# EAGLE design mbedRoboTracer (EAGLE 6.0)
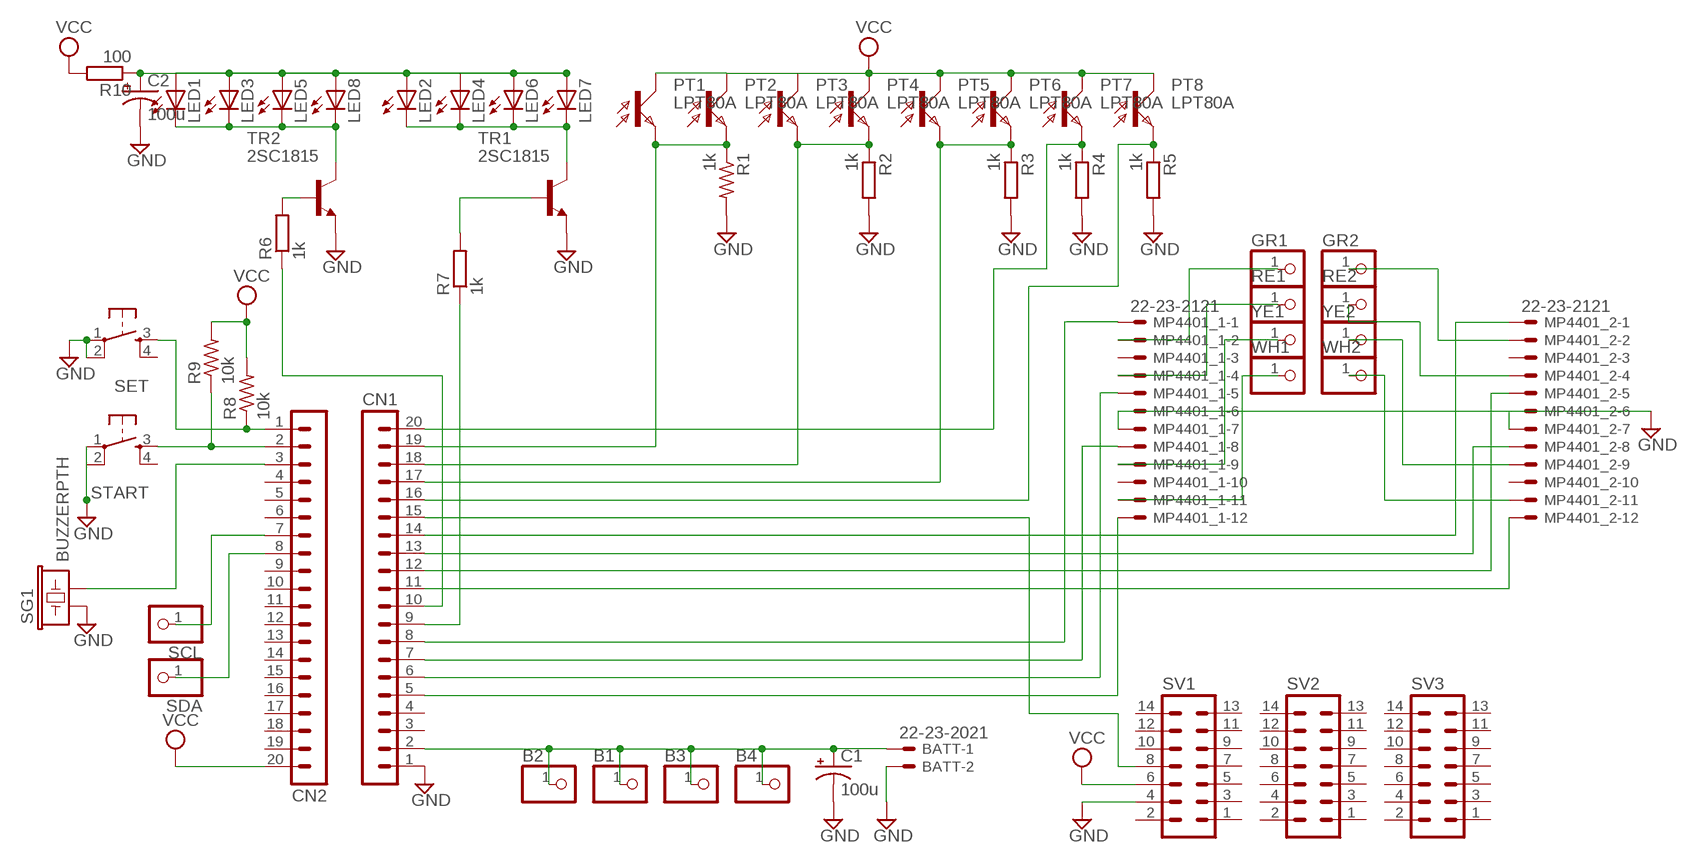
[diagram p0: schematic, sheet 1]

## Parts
B1  PINHD-1X1  [1X01]
B2  PINHD-1X1  [1X01]
B3  PINHD-1X1  [1X01]
B4  PINHD-1X1  [1X01]
BATT  22-23-2021  [22-23-2021]
C1  100u  CPOL-USTT2D5  [TT2D5]
C2  100u  CPOL-USTT2D5  [TT2D5]
CN1  MA20-1  [MA20-1]
CN2  MA20-1  [MA20-1]
GR1  PINHD-1X1  [1X01]
GR2  PINHD-1X1  [1X01]
LED1  LED3MM  [LED3MM]
LED2  LED3MM  [LED3MM]
LED3  LED3MM  [LED3MM]
LED4  LED3MM  [LED3MM]
LED5  LED3MM  [LED3MM]
LED6  LED3MM  [LED3MM]
LED7  LED3MM  [LED3MM]
LED8  LED3MM  [LED3MM]
MP4401_1  22-23-2121  [22-23-2121]
MP4401_2  22-23-2121  [22-23-2121]
PT1  LPT80A  [LPT80A]
PT2  LPT80A  [LPT80A]
PT3  LPT80A  [LPT80A]
PT4  LPT80A  [LPT80A]
PT5  LPT80A  [LPT80A]
PT6  LPT80A  [LPT80A]
PT7  LPT80A  [LPT80A]
PT8  LPT80A  [LPT80A]
R1  1k  R-US_0204/2V  [0204V]
R2  1k  R-EU_0204/2V  [0204V]
R3  1k  R-EU_0204/2V  [0204V]
R4  1k  R-EU_0204/2V  [0204V]
R5  1k  R-EU_0204/2V  [0204V]
R6  1k  R-EU_0204/2V  [0204V]
R7  1k  R-EU_0204/2V  [0204V]
R8  10k  R-US_0204/2V  [0204V]
R9  10k  R-US_0204/2V  [0204V]
R10  100  R-EU_0204/2V  [0204V]
RE1  PINHD-1X1  [1X01]
RE2  PINHD-1X1  [1X01]
SCL  PINHD-1X1  [1X01]
SDA  PINHD-1X1  [1X01]
SET  T-SWITCH-10  [B3F-10XX]
SG1  BUZZERPTH  [BUZZER-12MM]
START  T-SWITCH-10  [B3F-10XX]
SV1  MA07-2  [MA07-2]
SV2  MA07-2  [MA07-2]
SV3  MA07-2  [MA07-2]
TR1  2SC1815  [TO92-ECB]
TR2  2SC1815  [TO92-ECB]
WH1  PINHD-1X1  [1X01]
WH2  PINHD-1X1  [1X01]
YE1  PINHD-1X1  [1X01]
YE2  PINHD-1X1  [1X01]

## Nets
GND: BATT.2 C1.- C2.- CN1.1 MP4401_1.6 MP4401_1.7 MP4401_2.6 MP4401_2.7 R1.2 R2.2 R3.2 R4.2 R5.2 SET.1(P) SET.2(P1) SG1.+ START.1(P) START.2(P1) SV1.4 TR1.E TR2.E
N$1: CN1.17 PT5.E PT6.E R3.1
N$2: R7.2 TR1.B
N$3: CN1.8 MP4401_1.1
N$4: CN2.2 R9.1 START.3(S)
N$5: CN2.1 R8.1 SET.3(S)
N$6: CN1.15 SV1.8
N$7: LED1.K(C) LED3.K(C) LED5.K(C) LED8.K(C) TR2.C
N$8: CN1.18 PT3.E PT4.E R2.1
N$9: CN2.7 SCL.1
N$10: CN2.8 SDA.1
N$11: C2.+ LED1.A LED2.A LED3.A LED4.A LED5.A LED6.A LED7.A LED8.A R10.1
N$16: CN1.11 MP4401_2.12
N$17: CN1.6 MP4401_1.5
N$18: LED2.K(C) LED4.K(C) LED6.K(C) LED7.K(C) TR1.C
N$19: R6.2 TR2.B
N$20: CN2.3 SG1.-
N$21: CN1.20 PT7.E R4.1
N$22: CN1.9 R7.1
N$24: CN1.19 PT1.E PT2.E R1.1
N$25: B1.1 B2.1 B3.1 B4.1 BATT.1 C1.+ CN1.2
N$26: CN1.16 PT8.E R5.1
N$28: CN1.14 MP4401_2.1
N$29: CN1.10 R6.1
N$39: CN1.7 MP4401_1.8
N$41: CN1.12 MP4401_2.5
N$44: GR1.1 MP4401_1.2
N$45: MP4401_1.4 RE1.1
N$46: MP4401_1.11 WH1.1
N$47: CN1.5 MP4401_1.12
N$48: GR2.1 MP4401_2.2
N$49: MP4401_2.4 RE2.1
N$50: MP4401_2.9 YE2.1
N$51: MP4401_2.11 WH2.1
N$52: MP4401_1.9 YE1.1
N$61: CN1.13 MP4401_2.8
VCC: CN2.20 PT1.C PT2.C PT3.C PT4.C PT5.C PT6.C PT7.C PT8.C R8.2 R9.2 R10.2 SV1.6
Unconnected: CN1.3 CN1.4 CN2.4 CN2.5 CN2.6 CN2.9 CN2.10 CN2.11 CN2.12 CN2.13 CN2.14 CN2.15 CN2.16 CN2.17 CN2.18 CN2.19 MP4401_1.3 MP4401_1.10 MP4401_2.3 MP4401_2.10 SET.4(S1) START.4(S1) SV1.1 SV1.2 SV1.3 SV1.5 SV1.7 SV1.9 SV1.10 SV1.11 SV1.12 SV1.13 SV1.14 SV2.1 SV2.2 SV2.3 SV2.4 SV2.5 SV2.6 SV2.7 SV2.8 SV2.9 SV2.10 SV2.11 SV2.12 SV2.13 SV2.14 SV3.1 SV3.2 SV3.3 SV3.4 SV3.5 SV3.6 SV3.7 SV3.8 SV3.9 SV3.10 SV3.11 SV3.12 SV3.13 SV3.14

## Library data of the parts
B1-B4 GR1 GR2 RE1 RE2 SCL SDA WH1 WH2 YE1 YE2 = pinhead:PINHD-1X1: PIN HEADER
BATT = con-molex:22-23-2021: .100" (2.54mm) Center Header - 2 Pin
C1 C2 = resistor:CPOL-US: POLARIZED CAPACITOR, American symbol
CN1 CN2 = con-lstb:MA20-1: PIN HEADER; OC_FARNELL: unknown; OC_NEWARK: unknown
LED1-LED8 = led:LED: LED
MP4401_1 MP4401_2 = con-molex:22-23-2121: .100" (2.54mm) Center Header - 12 Pin
PT1-PT8 = opto-trans-siemens:LPT80A: PHOTO TRANSISTOR
R1 R8 R9 = resistor:R-US_: RESISTOR, American symbol
R2-R7 = rcl:R-EU_: RESISTOR, European symbol
R10 = resistor:R-EU_: RESISTOR, European symbol
SET START = 1-sw:T-SWITCH: TACTILE SWITCH
SG1 = SparkFun:BUZZER: Buzzer 12mm
SV1-SV3 = con-lstb:MA07-2: PIN HEADER; OC_FARNELL: unknown; OC_NEWARK: unknown
TR1 TR2 = transistor:2SC1815: NPN EPITAXIAL TRANSISTOR Source: TOSHIBA .. 2SC1815 1.pdf

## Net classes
1 +5V: width 0.61 mm, drill 0.406 mm
2 GND: width 0.914 mm, drill 0.406 mm

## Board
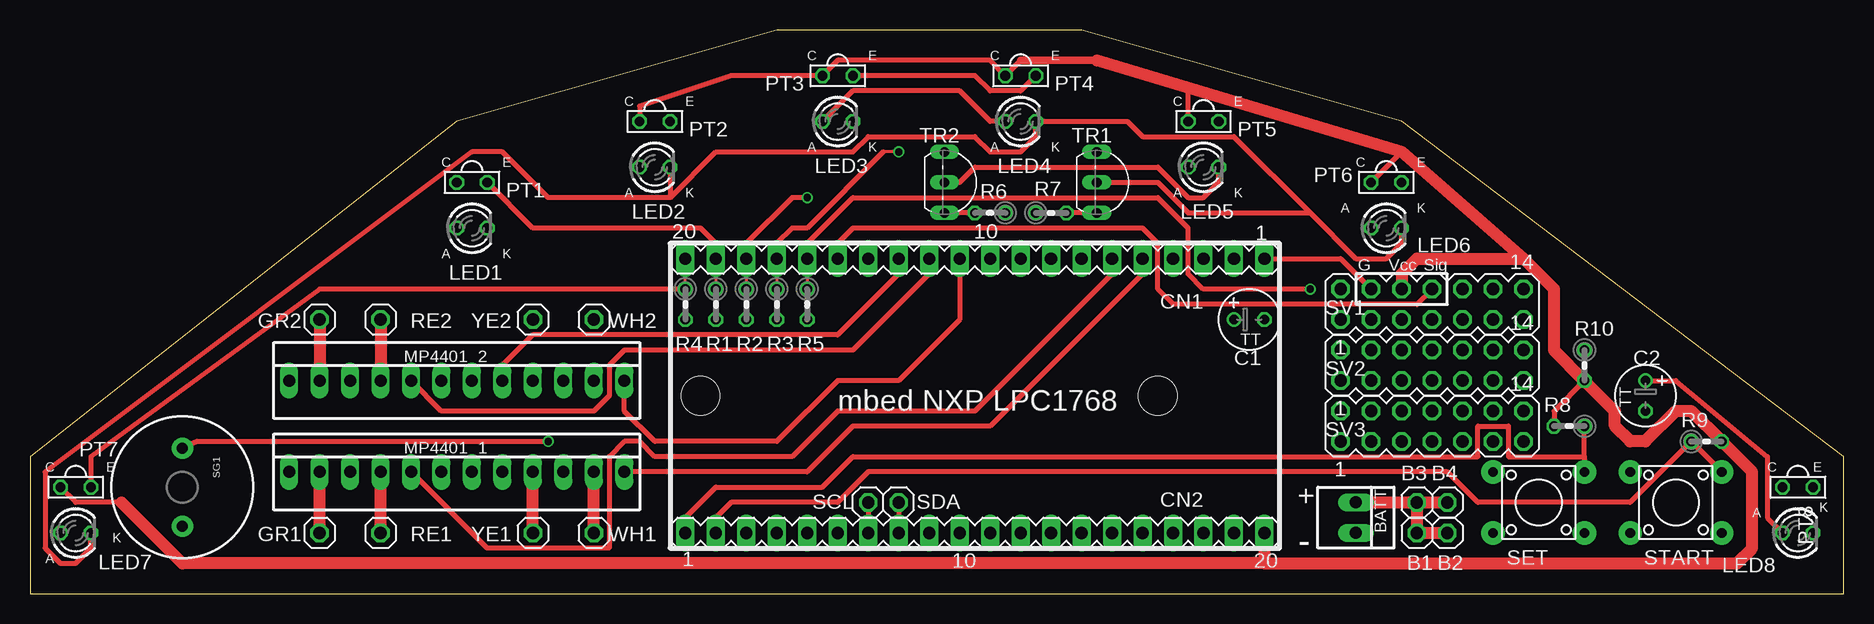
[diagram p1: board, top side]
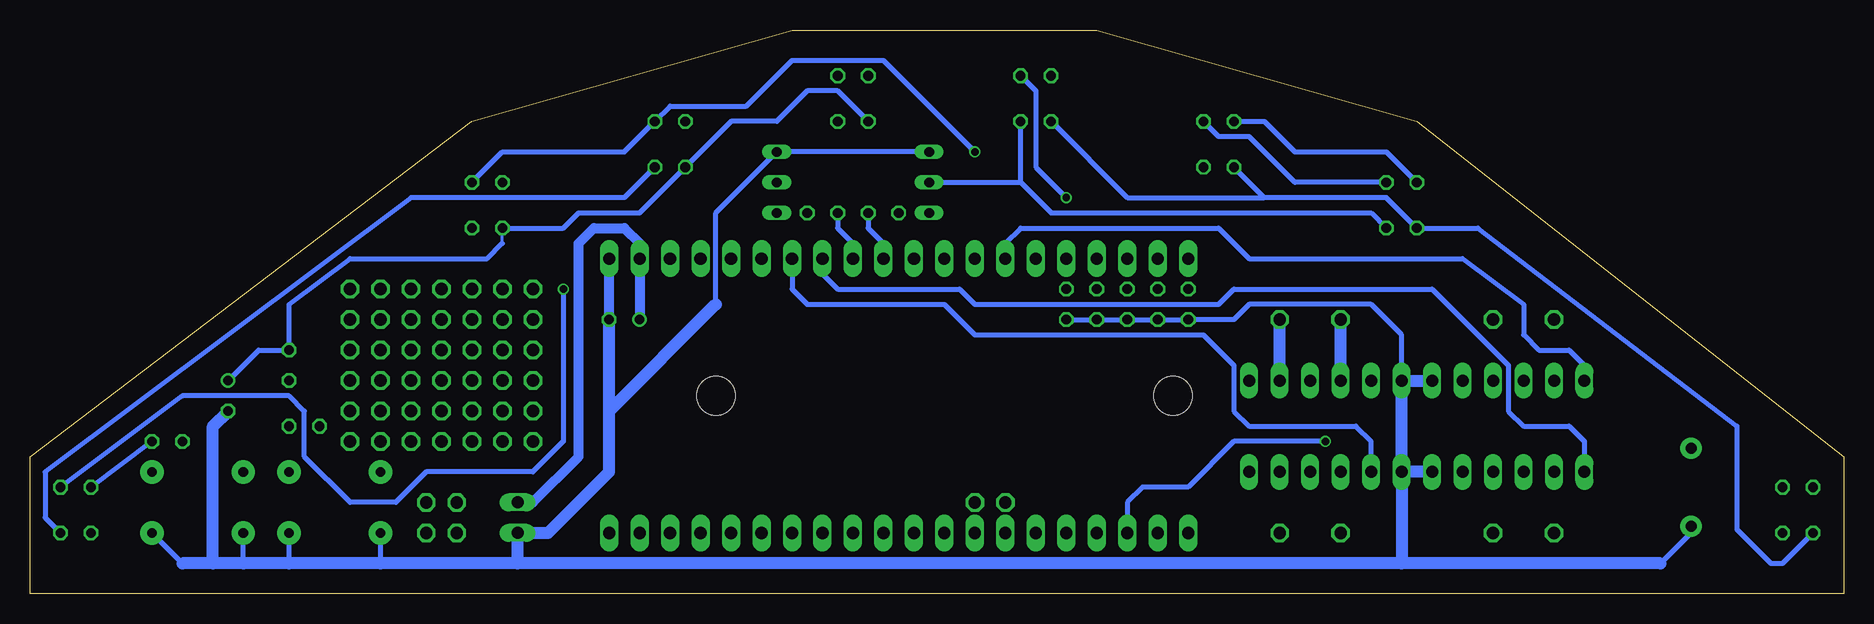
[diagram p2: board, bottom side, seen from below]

Size 151.13 x 46.99 mm. Coordinates in mm from the lower left corner, seen from the top.
Outline: 0,0 151.13,0 151.13,11.43 114.3,39.37 87.63,46.99 62.23,46.99 35.56,39.37 0,11.43 0,0
Copper layers (1*16): Top 0.035mm / dielectric 1.53mm / Bottom 0.035mm
Design rules: minimum track width 5mil, minimum drill 0.3mm, track to track 5mil, track to pad 0.229mm, pad to pad 5mil, via to via 5mil, smd to smd 5mil, copper to edge 0.5mm, drill to drill 0.5mm, minimum pad ring 0.15mm, minimum via ring 0.15mm, stop-mask expansion 4mil, vias tented up to drill 0.35mm, thermal gap 10mil
Holes 3.2 mm at 55.88,16.51 93.98,16.51

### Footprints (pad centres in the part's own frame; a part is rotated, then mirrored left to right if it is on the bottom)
1X01 = drill 1.016 octagon: 1 0,0
22-23-2021 = drill 1 long: 1 -1.27,0; 2 1.27,0
TT2D5 = drill 0.813: + -1.27,0 | drill 0.813 octagon: - 1.27,0
MA20-1 = drill 1.016 long: 1 -24.13,0; 2 -21.59,0; 3 -19.05,0; 4 -16.51,0; 5 -13.97,0; 6 -11.43,0; 7 -8.89,0; 8 -6.35,0; 9 -3.81,0; 10 -1.27,0; 11 1.27,0; 12 3.81,0; 13 6.35,0; 14 8.89,0; 15 11.43,0; 16 13.97,0; 17 16.51,0; 18 19.05,0; 19 21.59,0; 20 24.13,0
LED3MM = drill 0.813 octagon: A -1.27,0; K 1.27,0
22-23-2121 = drill 1 long: 1 -13.97,0; 2 -11.43,0; 3 -8.89,0; 4 -6.35,0; 5 -3.81,0; 6 -1.27,0; 7 1.27,0; 8 3.81,0; 9 6.35,0; 10 8.89,0; 11 11.43,0; 12 13.97,0
LPT80A = drill 0.813 octagon: C 0,-1.27; E 0,1.27
0204V = drill 0.813 octagon: 1 -1.27,0; 2 1.27,0
B3F-10XX = drill 0.813 pad 1.93: 1 -3.81,2.54; 2 3.81,2.54; 3 -3.81,-2.54; 4 3.81,-2.54
BUZZER-12MM = drill 0.9 pad 1.778: + 3.25,0; - -3.25,0
MA07-2 = drill 1.016 octagon: 1 -7.62,-1.27; 2 -7.62,1.27; 3 -5.08,-1.27; 4 -5.08,1.27; 5 -2.54,-1.27; 6 -2.54,1.27; 7 0,-1.27; 8 0,1.27; 9 2.54,-1.27; 10 2.54,1.27; 11 5.08,-1.27; 12 5.08,1.27; 13 7.62,-1.27; 14 7.62,1.27
TO92-ECB = drill 0.813 long: B 2.54,0; C 0,0; E -2.54,0

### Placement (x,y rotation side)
B1  115.57,5.08 0 top
B2  115.57,7.62 0 top
B3  118.11,7.62 0 top
B4  118.11,5.08 0 top
BATT  110.49,6.35 270 top
C1  101.6,22.86 0 top
C2  134.62,16.51 270 top
CN1  78.74,27.94 180 top
CN2  78.74,5.08 0 top
GR1  24.13,5.08 0 top
GR2  24.13,22.86 0 top
LED1  36.83,30.48 0 top
LED2  52.07,35.56 0 top
LED3  67.31,39.37 0 top
LED4  82.55,39.37 0 top
LED5  97.79,35.56 0 top
LED6  113.03,30.48 0 top
LED7  3.81,5.08 0 top
LED8  147.32,5.08 0 top
MP4401_1  35.56,10.16 0 top
MP4401_2  35.56,17.78 0 top
PT1  36.83,34.29 270 top
PT2  52.07,39.37 270 top
PT3  67.31,43.18 270 top
PT4  82.55,43.18 270 top
PT5  97.79,39.37 270 top
PT6  113.03,34.29 270 top
PT7  3.81,8.89 270 top
PT8  147.32,8.89 270 top
R1  57.15,24.13 270 top
R2  59.69,24.13 270 top
R3  62.23,24.13 270 top
R4  54.61,24.13 270 top
R5  64.77,24.13 270 top
R6  80.01,31.75 180 top
R7  85.09,31.75 0 top
R8  128.27,13.97 180 top
R9  139.7,12.7 0 top
R10  129.54,19.05 270 top
RE1  29.21,5.08 0 top
RE2  29.21,22.86 0 top
SCL  69.85,7.62 180 top
SDA  72.39,7.62 180 top
SET  125.73,7.62 180 top
SG1  12.7,8.89 270 top
START  137.16,7.62 180 top
SV1  116.84,24.13 0 top
SV2  116.84,19.05 0 top
SV3  116.84,13.97 0 top
TR1  88.9,34.29 270 top
TR2  76.2,34.29 270 top
WH1  46.99,5.08 0 top
WH2  46.99,22.86 0 top
YE1  41.91,5.08 0 top
YE2  41.91,22.86 0 top

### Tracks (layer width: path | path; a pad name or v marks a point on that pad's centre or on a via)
GND
  Top 0.406: CN1.1 109.22,27.94 SV1.4
  Bottom 0.406: SG1.+ 12.7,5.08 15.24,2.54 | 138.43,2.54 START.1 | 121.92,2.54 SET.2 | 129.54,2.54 SET.1 | 133.35,2.54 START.2 | MP4401_2.7 36.83,21.59 39.37,24.13 49.53,24.13 50.8,22.86 R4.2 R1.2 R2.2 R3.2 R5.2 | 93.98,24.13 93.98,31.75 TR1.E TR2.E
  Bottom 0.813: C1.- CN1.1
  Bottom 1.016: 102.87,15.24 102.87,10.16 107.95,5.08 BATT.2 110.49,2.54 | 102.87,15.24 C1.- | 15.24,2.54 36.83,2.54 | 36.83,2.54 110.49,2.54 | 110.49,2.54 121.92,2.54 129.54,2.54 133.35,2.54 135.89,2.54 | 135.89,2.54 138.43,2.54 | MP4401_1.7 36.83,2.54 | 102.87,15.24 93.98,24.13 | 135.89,2.54 135.89,13.97 C2.- | MP4401_2.6 MP4401_2.7 MP4401_1.7 | MP4401_1.6 MP4401_1.7
N$1  (via drill 0.61)
  Top 0.254: CN1.17 R3.1 | v72.39,36.83 71.12,36.83
  Top 0.406: 71.12,36.83 64.77,30.48 63.5,30.48 62.23,29.21 CN1.17
  Bottom 0.406: PT6.E 111.76,36.83 101.6,36.83 PT5.E 97.79,40.64 91.44,40.64 87.63,44.45 80.01,44.45 v72.39,36.83
N$2
  Top 0.406: TR1.B R7.2
N$3
  Bottom 0.254: CN1.8 85.09,26.67
  Bottom 0.406: MP4401_1.1 21.59,12.7 22.86,13.97 26.67,13.97 27.94,15.24 27.94,19.05 34.29,25.4 50.8,25.4 52.07,24.13 72.39,24.13 73.66,25.4 83.82,25.4 85.09,26.67
N$4
  Top 0.254: 57.15,6.35 CN2.2
  Top 0.406: START.3 R9.1 133.35,7.62 120.65,7.62 118.11,10.16 69.85,10.16 67.31,7.62 58.42,7.62 57.15,6.35
N$5
  Top 0.254: 54.61,6.35 CN2.1
  Top 0.406: 54.61,6.35 57.15,8.89 66.04,8.89 68.58,11.43 120.65,11.43 120.65,13.97 123.19,13.97 123.19,11.43 129.54,11.43 | 129.54,11.43 R8.1 | 129.54,11.43 SET.3
N$6
  Top 0.406: CN1.15 67.31,29.21 68.58,30.48 92.71,30.48 93.98,29.21 93.98,25.4 95.25,24.13 115.57,24.13 SV1.8
N$7
  Top 0.406: TR2.C 77.47,34.29 78.74,35.56 93.98,35.56 96.52,33.02 97.79,33.02 99.06,34.29 LED5.K
  Bottom 0.406: LED1.K 39.37,31.75 66.04,31.75 68.58,34.29 | TR2.C 68.58,34.29 | 68.58,34.29 LED3.K | LED5.K 101.6,33.02 119.38,33.02 149.86,10.16 149.86,6.35 LED8.K
N$8  (via drill 0.61)
  Top 0.254: CN1.18 R2.1
  Top 0.406: PT3.E 78.74,43.18 80.01,41.91 82.55,41.91 PT4.E | v64.77,33.02 63.5,33.02 59.69,29.21 CN1.18
  Bottom 0.406: v64.77,33.02 67.31,35.56 67.31,41.91 PT3.E
N$9
  Top 0.406: SCL.1 CN2.7
N$10
  Top 0.406: SDA.1 CN2.8
N$11
  Top 0.406: LED8.A 144.78,6.35 144.78,11.43 137.16,17.78 C2.+ | LED3.A 68.58,41.91 77.47,41.91 80.01,39.37 LED4.A
  Bottom 0.254: 111.76,29.21 LED6.A
  Bottom 0.406: 48.26,33.02 59.69,33.02 LED3.A | LED7.A 5.08,2.54 6.05,2.54 8.89,5.38 8.89,13.97 30.48,30.48 LED1.A 38.1,33.02 48.26,33.02 | 48.26,33.02 LED2.A | 111.76,29.21 113.03,27.94 124.46,27.94 129.54,24.13 R10.1 132.08,20.32 C2.+ | LED6.A 106.68,30.48 105.41,31.75 100.33,31.75 LED5.A 92.71,39.37 88.9,39.37 86.36,41.91 83.82,41.91 LED4.A
N$16
  Top 0.406: CN1.11 77.47,22.86 72.39,17.78 67.31,17.78 62.23,12.7 52.07,12.7 49.53,15.24 MP4401_2.12
N$17
  Top 0.406: MP4401_1.5 38.1,3.81 48.26,3.81 48.26,11.43 49.53,12.7 50.8,12.7 52.07,11.43 63.5,11.43 67.31,15.24 78.74,15.24 90.17,26.67 CN1.6
N$18
  Top 0.406: LED2.K 53.34,33.02 | 53.34,33.02 43.18,33.02 39.37,36.83 36.83,36.83 1.27,10.16 1.27,3.81 2.54,2.54 3.81,2.54 5.08,3.81 LED7.K | 53.34,33.02 57.15,36.83 68.58,36.83 69.85,38.1 78.74,38.1 80.01,36.83 82.55,36.83 83.82,38.1 LED4.K 91.44,39.37 92.71,38.1 100.33,38.1 106.68,31.75 | LED6.K 114.3,29.21 113.03,27.94 110.49,27.94 106.68,31.75 | TR1.C 93.98,34.29 96.52,31.75 106.68,31.75
N$19
  Top 0.406: R6.2 TR2.B
N$20  (via drill 0.61)
  Top 0.406: v43.18,12.7 13.97,12.7 SG1.-
  Bottom 0.406: v43.18,12.7 50.8,12.7 54.61,8.89 58.42,8.89 59.69,7.62 CN2.3
N$21
  Top 0.254: R4.1 CN1.20
  Top 0.406: PT7.E 5.08,11.43 24.13,25.4 R4.1
N$22
  Bottom 0.406: R7.1 83.82,30.48 82.55,29.21 CN1.9
N$24
  Top 0.254: CN1.19 R1.1
  Top 0.406: PT1.E 41.91,30.48 55.88,30.48 57.15,29.21 CN1.19
  Bottom 0.406: PT2.E 52.07,38.1 49.53,38.1 45.72,34.29 PT1.E
N$25
  Top 1.016: B2.1 B1.1 B4.1 | B2.1 B3.1 | BATT.1 B2.1
  Bottom 0.406: BATT.1 109.22,7.62
  Bottom 0.813: 109.22,7.62 105.41,11.43 105.41,29.21 104.14,30.48 101.6,30.48 100.33,29.21 CN1.2 C1.+
N$26  (via drill 0.61)
  Top 0.254: R5.1 CN1.16 64.77,29.21
  Top 0.406: v106.68,25.4 97.79,25.4 96.52,26.67 96.52,30.48 93.98,33.02 68.58,33.02 64.77,29.21
  Bottom 0.406: PT8.E 138.43,16.51 129.54,16.51 128.27,15.24 128.27,11.43 124.46,7.62 120.65,7.62 118.11,10.16 109.22,10.16 106.68,12.7 v106.68,25.4
N$28
  Bottom 0.254: CN1.14 69.85,29.21
  Bottom 0.406: MP4401_2.1 21.59,19.05 22.86,20.32 25.4,20.32 26.67,21.59 26.67,24.13 31.75,27.94 49.53,27.94 52.07,30.48 68.58,30.48 69.85,29.21
N$29
  Bottom 0.406: R6.1 81.28,30.48 80.01,29.21 CN1.10
N$39
  Bottom 0.406: CN1.7 87.63,25.4 86.36,24.13 74.93,24.13 72.39,21.59 53.34,21.59 50.8,19.05 50.8,15.24 49.53,13.97 40.64,13.97 39.37,12.7 MP4401_1.8
N$41
  Top 0.254: CN1.12 74.93,26.67
  Top 0.406: MP4401_2.5 34.29,15.24 46.99,15.24 48.26,16.51 48.26,19.05 49.53,20.32 68.58,20.32 74.93,26.67
N$44
  Top 1.016: GR1.1 MP4401_1.2
N$45
  Top 1.016: RE1.1 MP4401_1.4
N$46
  Top 1.016: WH1.1 MP4401_1.11
N$47
  Top 0.406: MP4401_1.12 64.77,10.16 68.58,13.97 80.01,13.97 92.71,26.67 CN1.5
N$48
  Top 1.016: GR2.1 MP4401_2.2
N$49
  Top 1.016: RE2.1 MP4401_2.4
N$50
  Bottom 1.016: MP4401_2.9 YE2.1
N$51
  Bottom 1.016: MP4401_2.11 WH2.1
N$52
  Top 1.016: YE1.1 MP4401_1.9
N$61
  Top 0.254: CN1.13 72.39,26.67
  Top 0.406: MP4401_2.8 39.37,19.05 41.91,21.59 67.31,21.59 72.39,26.67
VCC
  Top 0.406: 88.9,44.45 96.52,41.91 PT5.C | PT2.C 50.8,40.64 58.42,43.18 PT3.C 67.31,44.45 80.01,44.45 PT4.C 82.55,44.45 | PT7.C 3.81,7.62 7.62,7.62 | R10.2 127,15.24 R8.2 | 114.3,36.83 PT6.C
  Top 0.61: 82.55,44.45 88.9,44.45
  Top 1.016: CN2.20 102.87,2.54 | 7.62,7.62 12.7,2.54 102.87,2.54 | 102.87,2.54 142.24,2.54 143.51,3.81 143.51,10.16 R9.2 138.43,15.24 137.16,15.24 134.62,12.7 133.35,12.7 132.08,13.97 132.08,15.24 R10.2 127,20.32 127,25.4 124.46,27.94 | 88.9,44.45 114.3,36.83 124.46,27.94 | 124.46,27.94 115.57,27.94 114.3,26.67 SV1.6
  Bottom 0.406: PT1.C 38.1,36.83 45.72,36.83 48.26,39.37 PT2.C | PT8.C R9.2

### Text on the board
tPlace: C | E | C | E | C | E | C | E | A | K | A | K | C | E | C | E | A | K | A | K | A | K | A | K | G | Vcc | Sig | C | E | C | E | + | K | - | A | K | A
tNames: mbed NXP LPC1768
